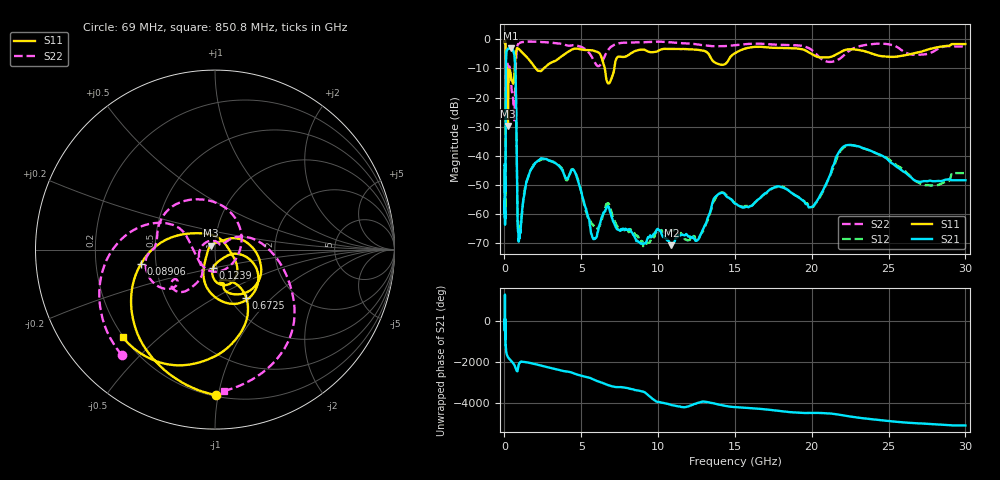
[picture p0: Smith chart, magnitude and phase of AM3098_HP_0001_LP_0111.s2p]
! Date/Time: Thu, Feb 28, 2019 8:31 AM
! Network Analyzer: Agilent Technologies E8364B Rev: A.07.50.67
! Sweep from 0.010 to 30.000 GHz, 1601 Points, Sweep Type: LOG
! Power Supply: 5.022 V, 0.002 A
# Hz S DB R 50
!freq MagS11 AngS11 MagS21 AngS21 MagS12 AngS12 MagS22 AngS22
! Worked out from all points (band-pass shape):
!   1601 points, 10 MHz to 30 GHz, reference 50 ohm
!   highest |S21| = -3.10 dB at 418 MHz (marker M1); lowest = -70.8 dB at 10.86 GHz (marker M2)
!   |S21| within 3 dB of the highest: 104.6 MHz to 660.5 MHz (556 MHz wide, 145 % of centre)
!   lowest |S11| = -29.8 dB at 225.9 MHz (marker M3), VSWR 1.07, Z = 47.7 + j2.17 ohm
!   |S11| at or under -10 dB: 175.8 MHz to 671.1 MHz (495.4 MHz wide, 117 % of centre); 2.041 GHz to 2.551 GHz (510.8 MHz wide, 22.2 % of centre); 6.529 GHz to 7.149 GHz (620.1 MHz wide, 9.07 % of centre)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
!   |S22| runs from -28.2 to -0.6 dB; largest |S21 - S12| = 0.01
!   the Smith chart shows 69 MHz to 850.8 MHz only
!   S11 on the Smith chart (normalised r, x): 69 MHz: 0.21, -0.99; 89.06 MHz: 0.41, -0.08; 123.9 MHz: 0.96, -0.20; 672.5 MHz: 1.19, -0.71; 850.8 MHz: 0.20, -0.39
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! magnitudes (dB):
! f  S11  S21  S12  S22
! 10 MHz  -0.4  -43.1  -45.2  -0.6
! 38.04 MHz  -0.5  -60.0  -60.8  -0.9
! 69 MHz  -1.8  -51.3  -51.8  -2.1
! 89.06 MHz  -7.5  -19.8  -19.8  -8.7
! 98.93 MHz  -23.8  -7.8  -7.8  -16.9
! 123.9 MHz  -19.7  -4.3  -4.3  -10.6
! 144.7 MHz  -13.2  -3.7  -3.6  -10.1
! 225.9 MHz  -29.8  -3.2  -3.2  -9.4
! 418 MHz  -12.5  -3.1  -3.1  -13.2
! 550.5 MHz  -15.1  -3.8  -3.7  -19.3
! 672.5 MHz  -9.9  -6.8  -6.7  -23.5
! 743.2 MHz  -5.0  -16.8  -16.8  -8.4
! 850.8 MHz  -3.0  -60.7  -61.0  -2.1
! 959.3 MHz  -3.4  -67.9  -66.5  -1.3
! 2.084 GHz  -10.3  -42.1  -42.3  -0.8
! 4.503 GHz  -3.3  -45.0  -44.8  -2.0
! 5.783 GHz  -3.8  -68.7  -64.0  -6.9
! 7.926 GHz  -5.8  -65.5  -65.8  -1.1
! 10.86 GHz  -3.2  -70.8  -65.7  -1.0
! 20 GHz  -5.1  -57.7  -57.6  -3.6
! 22.67 GHz  -3.4  -36.4  -36.4  -3.2
! 30 GHz  -1.6  -48.5  -46.0  -2.4
